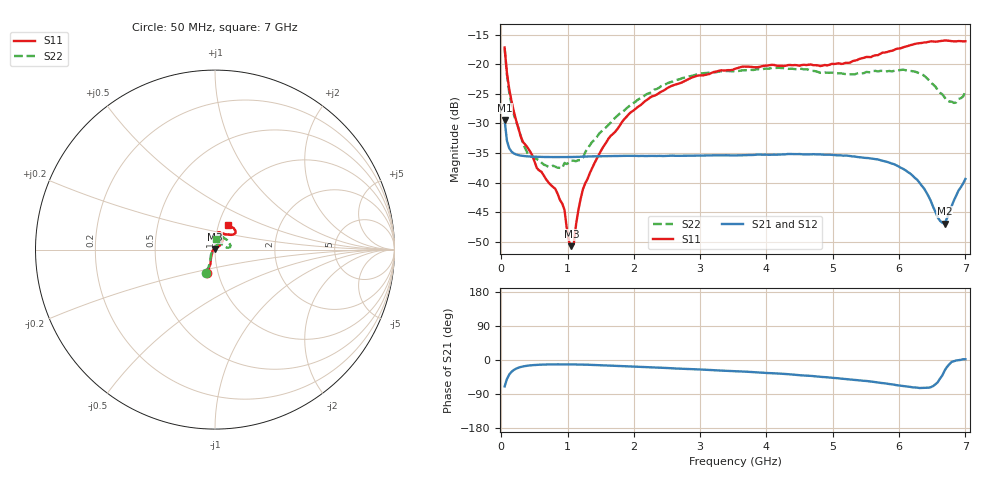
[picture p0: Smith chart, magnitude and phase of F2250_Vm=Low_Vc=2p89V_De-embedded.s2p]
! Integrated Device Technology
! Corporate Headquarters
! 6024 Silver Creek Valley Road
! San Jose, CA 95138  USA
! Phone:  1-408-284-8200
! Toll Free:  1-800-223-1366
! Webpage:  http://www.idt.com/
! Timing and RF Division
! 515 Groton Road, Suite 102
! Westford, MA 01886-6024
! Device:  F2250
! Description: Voltage Variable RF Attenuator
! Frequency:  50.0 -  6000.00 MHz
! Package:  3x3 mm Thin QFN Plastic Package: 16 pin
! Ports:  2 RF, 3 DC
!  Pin  1  = GND
!  Pin  2  = NC
!  Pin  3  = RF1  = Port 1
!  Pin  4  = NC
!  Pin  5  = GND
!  Pin  6  = GND
!  Pin  7  = GND
!  Pin  8  = GND
!  Pin  9  = NC
!  Pin 10  = RF2  = Port 2
!  Pin 11  = NC
!  Pin 12  = GND
!  Pin 13  = GND
!  Pin 14  = VCNTRL
!  Pin 15  = VDD
!  Pin 16  = VMODE
! Vcntrl:  2.890 Volts
! Vmode:  +0.000 Volts
! Vdd:  +3.30  Volts
! Current:  1.176 mA
! Data:  The device was measured on a the F2250 evaluation board which has
!  individual transmission lines to the RF pins.  Data was collected
!  using a calibrated network analyzer.  The evaluation board was
!  de-embedded using a TRL calibration technique.
!  The reference plane is the edge of the package pin.
! Misc:  SN 10
!  Action Tracker AT0258
! Date Measured:  2014-11-26
! Date:  2015-10-15  MJV
! Note:
!  Integrated Device Technology supplies this data as a sample of measured
!  data at the package pin for this product.  Your particular data for this
!  product may vary.
!  Data was taken at 25 degrees C.
!  Integrated Device Technology reserves the right to change this data at anytime.
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# GHz S dB R 50
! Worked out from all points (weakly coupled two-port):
!   201 points, 50 MHz to 7 GHz, reference 50 ohm
!   highest |S21| = -29.42 dB at 50 MHz (marker M1); lowest = -46.9 dB at 6.687 GHz (marker M2)
!   lowest |S11| = -50.7 dB at 1.058 GHz (marker M3), VSWR 1.01, Z = 49.8 + j0.243 ohm
!   |S11| at or under -10 dB: start of sweep to end of sweep
!   |S22| runs from -37.6 to -17.3 dB; largest |S21 - S12| = 6.4e-05
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0.05  -17.18 -108.6  -29.42 -69.8  -29.42 -69.8  -17.27 -111.0
0.08475  -21.45 -107.5  -32.92 -50.4  -32.92 -50.3  -21.74 -110.2
0.15425  -26.23 -116.6  -34.76 -31.2  -34.76 -31.1  -26.81 -122.4
0.29325  -32.21 -127.9  -35.43 -18.5  -35.43 -18.5  -32.09 -137.3
0.3975  -34.10 -141.8  -35.56 -15.0  -35.56 -15.0  -35.06 -160.4
0.91875  -43.52 158.0  -35.69 -11.5  -35.68 -11.5  -37.56 133.5
0.9535  -44.60 169.9  -35.69 -11.5  -35.68 -11.5  -36.67 131.1
1.023  -49.99 143.4  -35.68 -11.6  -35.67 -11.6  -36.64 115.9
1.05775  -50.72 123.1  -35.67 -11.6  -35.67 -11.6  -36.27 110.6
1.0925  -50.40 89.5  -35.66 -11.7  -35.65 -11.7  -36.30 106.5
1.162  -44.66 56.9  -35.64 -11.9  -35.64 -11.9  -36.20 95.5
1.2315  -41.11 44.3  -35.61 -12.1  -35.61 -12.1  -35.81 85.6
1.6485  -32.11 41.9  -35.52 -14.6  -35.52 -14.6  -29.88 64.5
1.9265  -28.40 41.3  -35.47 -16.9  -35.47 -16.9  -27.10 56.7
2.37825  -24.87 47.3  -35.48 -20.3  -35.48 -20.3  -23.98 56.8
3.525  -20.79 72.5  -35.40 -29.5  -35.40 -29.5  -21.19 74.7
4.7065  -20.17 72.3  -35.19 -42.6  -35.19 -42.6  -21.14 72.2
5.85325  -17.81 40.5  -36.63 -63.4  -36.63 -63.5  -21.14 23.1
6.27025  -16.50 40.0  -39.49 -72.8  -39.50 -72.9  -21.37 9.7
6.68725  -15.99 48.7  -46.89 -27.8  -46.89 -27.5  -25.63 28.6
6.861  -16.14 55.1  -42.20 -1.3  -42.15 -1.3  -26.45 57.9
7  -16.13 63.2  -39.37 1.9  -39.33 1.7  -24.63 83.1
